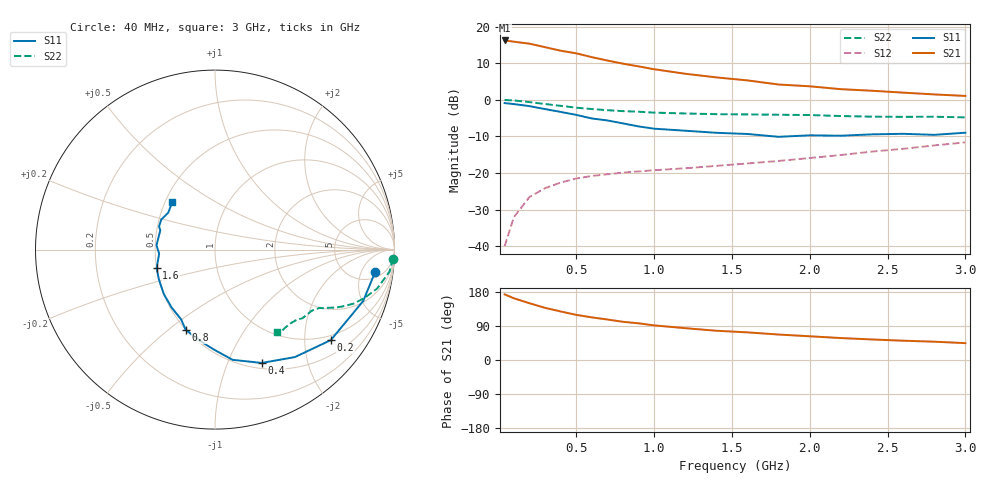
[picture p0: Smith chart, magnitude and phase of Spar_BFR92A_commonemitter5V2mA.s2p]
! Filename:  BFR92AA.S2P  Version:  2.0
! NXP part #: BFR92A  Date: May 1990
! Bias condition: Vce=5V, Ic=2mA
#  MHz  S  MA  R  50
! Freq  S11  S21  S12  S22  !GUM [dB]
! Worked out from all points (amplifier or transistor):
!   21 points, 40 MHz to 3 GHz, reference 50 ohm
!   highest |S21| = 16.2 dB at 40 MHz (marker M1)
!   |S21| within 3 dB of that: start of sweep to 427 MHz
!   unconditionally stable (mu >= 1): 1.565 GHz to 2.87 GHz
!   at 300 MHz: K = 0.29, MSG = 19.3 dB, |S12| = -24.2 dB
!   at 1 GHz: K = 0.81, MSG = 13.8 dB, |S12| = -19.3 dB
!   at 3 GHz: K = 0.98, MSG = 6.3 dB, |S12| = -11.6 dB
!   S11 on the Smith chart (normalised r, x): 40 MHz: 7, -9; 200 MHz: 0.87, -2.65; 400 MHz: 0.56, -1.34; 800 MHz: 0.50, -0.58; 1.6 GHz: 0.50, -0.12; 3 GHz: 0.55, +0.33
40  0.901 -7.9  6.467 173.2  0.01 86.1  0.994 -2.9
100  0.874 -19.1  6.222 162.8  0.025 78.1  0.979 -7.3
200  0.819 -38.0  5.842 149.8  0.047 70.8  0.93 -13.4
300  0.746 -53.4  5.235 137.6  0.062 64.0  0.875 -18.0
400  0.683 -67.6  4.679 128.1  0.074 58.8  0.827 -21.4
500  0.622 -80.9  4.317 119.1  0.084 55.7  0.78 -23.9
600  0.556 -90.8  3.824 112.5  0.091 53.5  0.747 -25.6
700  0.522 -97.7  3.441 106.9  0.096 53.0  0.721 -26.7
800  0.476 -110.1  3.116 100.8  0.101 52.4  0.7 -27.6
900  0.433 -115.7  2.863 96.8  0.105 53.4  0.687 -28.4
1000  0.403 -126.9  2.615 91.4  0.109 54.5  0.668 -29.1
1200  0.378 -138.9  2.269 84.0  0.116 56.2  0.65 -30.7
1400  0.354 -152.1  2.023 77.2  0.125 58.8  0.636 -32.6
1600  0.341 -162.5  1.84 72.9  0.135 62.8  0.631 -34.3
1800  0.312 -175.7  1.617 67.2  0.146 66.2  0.625 -36.2
2000  0.327 175.7  1.529 62.6  0.16 68.7  0.619 -38.2
2200  0.323 160.6  1.397 57.9  0.176 71.3  0.6 -40.6
2400  0.337 157.7  1.329 54.2  0.196 72.5  0.588 -44.4
2600  0.343 150.9  1.253 50.9  0.214 74.1  0.585 -48.0
2800  0.332 141.7  1.184 48.3  0.238 75.0  0.587 -50.8
3000  0.355 132.2  1.129 44.5  0.262 74.7  0.575 -53.1
